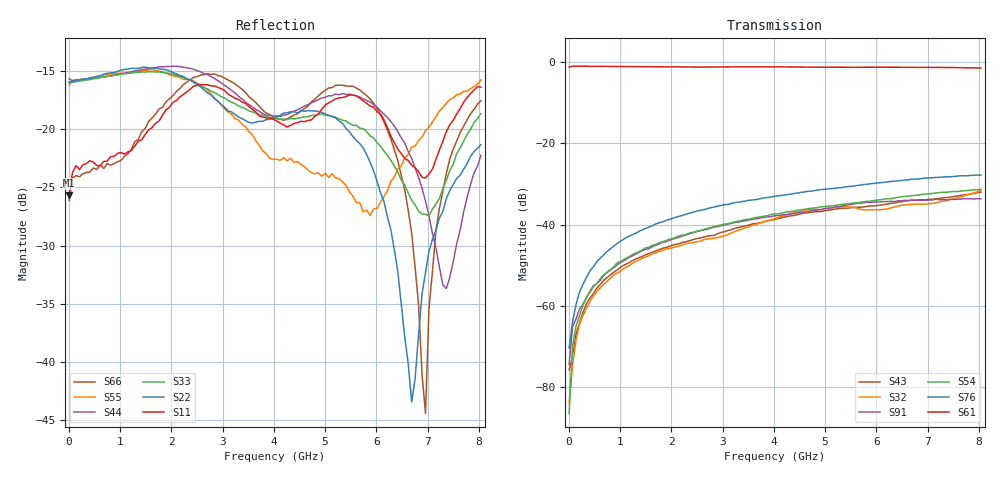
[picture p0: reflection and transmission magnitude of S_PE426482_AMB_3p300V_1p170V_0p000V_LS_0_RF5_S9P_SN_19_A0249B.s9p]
! Device ID: PE426482
! File Path: z:\PE426482\Final Char Data\room\AMB\3p300\LS_0_RF5\PE426482_AMB_3p300V_1p170V_0p000V_LS_0_RF5_S9P_SN_19_A0249B.s9p
! Serial: 19
! Lot: A0249B
! Temp: AMB
! VDD: 3.300
! VSS: 0.000
! Control_Hi: 1.170
! Control_Lo: 0.000
! Logic State: LS_0_RF5
! Port 1:
! Port 2:
! Port 3:
! Port 4:
! Port 5:
! Port 6:
! Port 7:
! Port 8:
! Port 9:
! ThroughPath:1-6
! IDD: 0.000107434
! ISS/IDD2: -7.15e-008
! IDMM3/IDD3: -2.307e-007
! Comment:
#  Hz  S  RI  R  50
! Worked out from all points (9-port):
!   120 points, 10 MHz to 8.037 GHz, reference 50 ohm
!   strongest paths, dB at 10 MHz, 2.034 GHz, 4.057 GHz, 6.08 GHz, 8.037 GHz:
!     S61: -1.2, -1.1, -1.1, -1.2, -1.4
!     S76: -70.4, -38.4, -33.0, -29.7, -27.8
!     S54: -86.5, -43.4, -37.4, -33.9, -31.3
!     S91: -74.5, -43.6, -37.8, -34.4, -33.7
!     S32: -83.9, -45.7, -38.4, -36.3, -31.6
!     S43: -75.8, -45.1, -38.6, -35.2, -32.0
!   lowest |S11| = -25.7 dB at 10 MHz (marker M1), VSWR 1.11, Z = 54.3 - j3.26 ohm
!   |S11| at or under -10 dB: start of sweep to end of sweep
